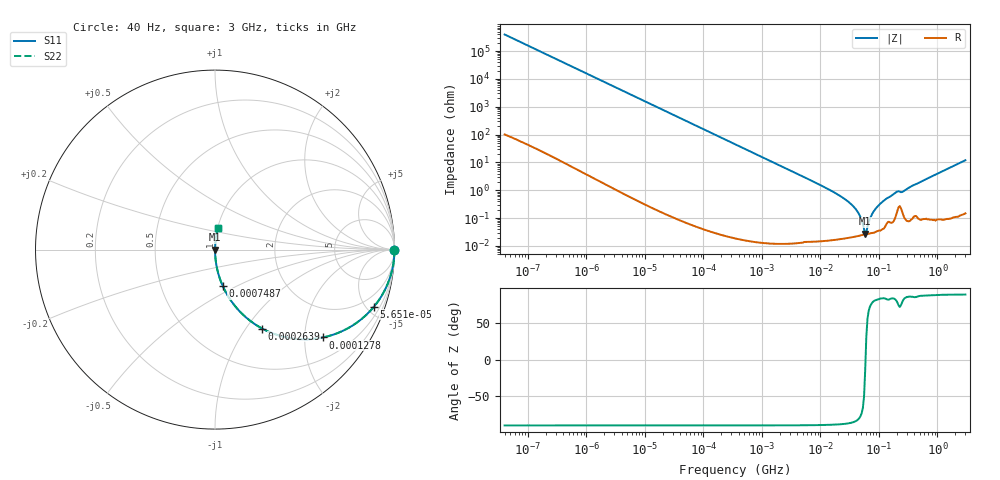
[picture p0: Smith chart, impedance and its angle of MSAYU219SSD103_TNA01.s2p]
! MSAYU219SSD103_TNA01  S-PARAMETER MODEL  ( General Type )
! Model Generated by TAIYO YUDEN Corporation (http://www.ty-top.com)
! Version 2.0
! TAIYO YUDEN Control No. 031016
! Copyright(c) 2003 TAIYO YUDEN CO.,LTD. All Rights Reserved.
! Product Description (link to TY-COMPAS)
! https://ds.yuden.co.jp/TYCOMPAS/or/detail?pn=MSAYU219SSD103KTNA01&u=M
! Products Name : Multilayer Ceramic Capacitors
! Characteristics :
!  Capacitance : 0.01 uF , Rated Voltage : 50V
!  Case Size : 2.0 x 1.25 / 0.079 x 0.049 [mm/inch] , Thickness : 0.85 / 0.033 [mm/inch]
!  (Conditions: Temperature = 25 degC , DC Bias Current/Voltage = 0A / 0V)
! External Node Assignments :
!  1  o---| |---o  2
! GND o---------o GND
! Frequency Range : 40Hz  -  3GHz  [ 401 STEP ]
# MHz S RI R 50
! Freq[MHz].  S11 Real  S11 Imag  S21 Real  S21 Imag  S12 Real  S12 Imag  S22 Real  S22 Imag
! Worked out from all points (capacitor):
!   401 points, 40 Hz to 3 GHz, reference 50 ohm
!   read as one part in series: C = 10.1 nF near 44 Hz
!   lowest |Z| = 27.5 mohm at 58.12 MHz (marker M1)
!   series resonance near 58.92 MHz, so ESL is about 720 pH
!   S11 on the Smith chart (normalised r, x): 40 Hz: open; 56.51 kHz: 1.00, -5.57; 127.8 kHz: 1.00, -2.46; 263.9 kHz: 1.00, -1.19; 748.7 kHz: 1.00, -0.42; 3 GHz: 1.00, +0.24
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4e-05  1 -0.000254  1.3e-07 0.000254  1.3e-07 0.000254  1 -0.000254
0.000834  1 -0.0053  2.93e-05 0.0053  2.93e-05 0.0053  1 -0.0053
0.017386  0.9879 -0.1091  0.0121 0.1091  0.0121 0.1091  0.9879 -0.1091
0.056505  0.8858 -0.318  0.1142 0.318  0.1142 0.318  0.8858 -0.318
0.12778  0.6027 -0.4892  0.3973 0.4892  0.3973 0.4892  0.6027 -0.4892
0.263915  0.2625 -0.4398  0.7375 0.4398  0.7375 0.4398  0.2625 -0.4398
0.362475  0.1588 -0.3652  0.8412 0.3652  0.8412 0.3652  0.1588 -0.3652
0.748653  0.0424 -0.2013  0.9576 0.2013  0.9576 0.2013  0.0424 -0.2013
1.939641  0.00664 -0.0805  0.9934 0.0805  0.9934 0.0805  0.00664 -0.0805
7.222098  0.000602 -0.0215  0.9994 0.0215  0.9994 0.0215  0.000602 -0.0215
18.71131  0.000225 -0.00754  0.9998 0.00754  0.9998 0.00754  0.000225 -0.00754
32.2371  0.000211 -0.0034  0.9998 0.0034  0.9998 0.0034  0.000211 -0.0034
44.27611  0.00023 -0.00154  0.9998 0.00154  0.9998 0.00154  0.00023 -0.00154
55.54024  0.000258 -0.000319  0.9997 0.000319  0.9997 0.000319  0.000258 -0.000319
58.11596  0.000265 -7.13e-05  0.9997 7.13e-05  0.9997 7.13e-05  0.000265 -7.13e-05
63.63129  0.000268 0.000397  0.9997 -0.000397  0.9997 -0.000397  0.000268 0.000397
72.90103  0.000289 0.00111  0.9997 -0.00111  0.9997 -0.00111  0.000289 0.00111
87.39454  0.000322 0.00214  0.9997 -0.00214  0.9997 -0.00214  0.000322 0.00214
150.5692  0.00076 0.00562  0.9992 -0.00562  0.9992 -0.00562  0.00076 0.00562
197.6342  0.0014 0.00844  0.9986 -0.00844  0.9986 -0.00844  0.0014 0.00844
259.4108  0.00139 0.00895  0.9986 -0.00895  0.9986 -0.00895  0.00139 0.00895
3000  0.0156 0.1179  0.9844 -0.1179  0.9844 -0.1179  0.0156 0.1179
